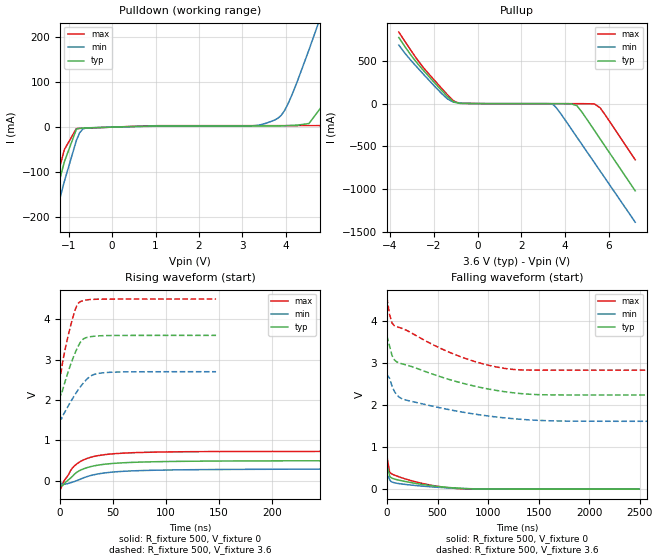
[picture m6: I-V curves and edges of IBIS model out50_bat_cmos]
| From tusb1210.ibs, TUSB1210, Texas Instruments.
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|   Model: out50_bat_cmos
|   Description:  Output buffer under VBAT NMOS/PMOS enabled
[Model]   out50_bat_cmos
Model_type   Output
Polarity   Non-Inverting
Vmeas =   1.800
Vref =   0
Cref =   5e-12
Rref =   10e9
|variable   typ   min   max
C_comp   0.087p   0.067p   0.184p
[Temperature Range]   27   125   -40
[Voltage Range]   3.6   2.7   4.5
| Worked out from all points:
|   slope of the pulldown table from 0 to 0.54 V, typ, clamps not added: 348 ohm
|   slope of the pullup table from 0 to 0.54 V, typ, clamps not added: 570 ohm
|   rising waveform, R_fixture 500, V_fixture 0: 20-80 % time 27.2ns typ, 38.7ns min, 21.3ns max; typ from 0 V to 0.494 V
|   rising waveform, R_fixture 500, V_fixture 3.6: 20-80 % time 11.6ns typ, 16.8ns min, 9.37ns max; typ from 2.25 V to 3.6 V
|   falling waveform, R_fixture 500, V_fixture 0: 20-80 % time 371ns typ, 397ns min, 321ns max; typ from 0.495 V to 0 V
|   falling waveform, R_fixture 500, V_fixture 3.6: 20-80 % time 730ns typ, 707ns min, 689ns max; typ from 3.6 V to 2.25 V
[Pulldown]
| out50_bat_cmos
|Voltage   I(typ)   I(min)   I(max)
-3.6V     -1.024A    -1.054A    -1.006A
-1.657V   -284.2mA   -326.4mA   -257.6mA
-1.38V    -178.7mA   -222.5mA   -151.2mA
-825mV    -4.513mA   -29.35mA   -3.185mA
3.675V    2.714mA    12.97mA    3.328mA
3.975V    2.963mA    36.45mA    3.331mA
4.541V    8.028mA    171.5mA    3.34mA
4.807V    42.23mA    243.7mA    3.391mA
5.339V    181.9mA    391.8mA    6.359mA
5.604V    256.7mA    467mA      34.86mA
6.402V    488.4mA    724.8mA    255.5mA
7.2V      776.3mA    1.027A     498.3mA
[Pullup]
| out50_bat_cmos
|Voltage   I(typ)   I(min)   I(max)
-3.6V     774mA      686mA      837.8mA
-3.045V   567.2mA    505.7mA    622.9mA
-2.49V    393.2mA    348.2mA    425.5mA
-1.38V    82.25mA    54.58mA    104mA
-1.103V   19.41mA    16.33mA    31.43mA
-825mV    2.848mA    5.981mA    3.142mA
3.45V     -989.9uA   -12.69mA   -1.452mA
4.275V    -2.542mA   -296mA     -1.453mA
4.541V    -25.44mA   -395.5mA   -1.454mA
5.339V    -315.9mA   -693.7mA   -4.336mA
5.604V    -417mA     -793.2mA   -51.5mA
7.2V      -1.023A    -1.391A    -658.6mA
[Ramp]
| out50_bat_cmos
|variable   typ   min   max
dV/dt_r   0.495/2.724e-08   0.292/3.991e-08   0.726/2.128e-08
dV/dt_f   1.355/7.311e-07   1.082/7.070e-07   1.662/6.895e-07
R_load =   50
[Rising Waveform]
| out50_bat_cmos
R_fixture =   500
V_fixture =   0
V_fixture_min =   0
V_fixture_max =   0
|Time   V(typ)   V(min)   V(max)
0s        3.599uV    8.232uV    4.822uV
533.3ps   -133mV     -67.61mV   -210.4mV
2.386ns   -121mV     -94.18mV   -71.31mV
4.238ns   -65.07mV   -87.23mV   17.62mV
11.65ns   109mV      -36.2mV    316.1mV
20.91ns   280.2mV    57.26mV    500.2mV
32.02ns   367mV      147.4mV    600.5mV
50.54ns   428.4mV    215.3mV    666.7mV
126.5ns   482.2mV    272.2mV    718.6mV
367.5ns   494.3mV    290mV      725.8mV
[Rising Waveform]
| out50_bat_cmos
R_fixture =   500
V_fixture =   3.6
V_fixture_min =   2.7
V_fixture_max =   4.5
|Time   V(typ)   V(min)   V(max)
0s        2.245V     1.618V     2.838V
521.2ps   2.123V     1.557V     2.64V
1.262ns   2.139V     1.529V     2.751V
4.964ns   2.482V     1.728V     3.288V
10.89ns   2.95V      1.998V     3.94V
15.33ns   3.237V     2.185V     4.312V
19.03ns   3.425V     2.324V     4.435V
29.4ns    3.57V      2.602V     4.49V
39.03ns   3.591V     2.668V     4.498V
147.2ns   3.6V       2.7V       4.5V
[Falling Waveform]
| out50_bat_cmos
R_fixture =   500
V_fixture =   0
V_fixture_min =   0
V_fixture_max =   0
|Time   V(typ)   V(min)   V(max)
0s        494.6mV    292.3mV    726.2mV
1.068ns   528.9mV    316.7mV    767.6mV
13.65ns   456.1mV    304.3mV    582mV
26.23ns   310.4mV    224mV      407.9mV
51.4ns    260.3mV    169.3mV    358.7mV
290.5ns   135mV      85.46mV    170.7mV
579.9ns   46.36mV    33.87mV    41.65mV
743.5ns   17.7mV     16.6mV     7.763mV
949.4ns   2.653mV    5.3mV      373.1uV
2.494us   3.808uV    8.52uV     5.048uV
[Falling Waveform]
| out50_bat_cmos
R_fixture =   500
V_fixture =   3.6
V_fixture_min =   2.7
V_fixture_max =   4.5
|Time   V(typ)   V(min)   V(max)
0s        3.6V       2.7V       4.5V
25.39ns   3.418V     2.643V     4.168V
49.18ns   3.191V     2.466V     3.962V
72.97ns   3.083V     2.332V     3.898V
120.5ns   3.009V     2.194V     3.855V
215.7ns   2.945V     2.108V     3.761V
691.5ns   2.563V     1.861V     3.192V
1.167us   2.323V     1.699V     2.878V
1.643us   2.247V     1.629V     2.838V
4.715us   2.245V     1.618V     2.838V
